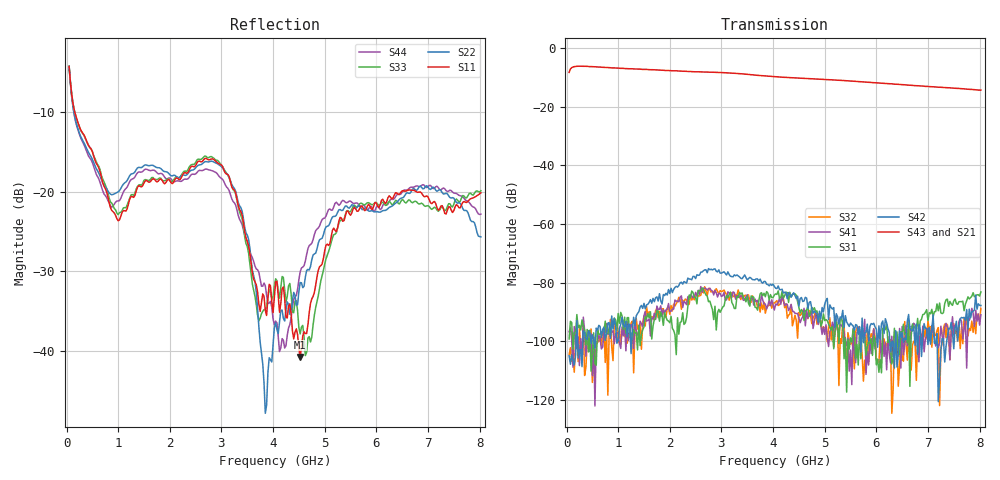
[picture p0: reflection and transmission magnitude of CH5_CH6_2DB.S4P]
!Agilent Technologies,E5071C,MY46316741,A.11.02
!Date: Mon Jun 01 10:40:18 2026
!Data & Calibration Information:
!1:CH5 INPUT 2:CH5 OUTPUT 3:CH6 INPUT 4:CH6 OUTPUT
!Freq	S11:SOLT4(ON)	S12:SOLT4(ON)	S13:SOLT4(ON)	S14:SOLT4(ON)
!	S21:SOLT4(ON)	S22:SOLT4(ON)	S23:SOLT4(ON)	S24:SOLT4(ON)
!	S31:SOLT4(ON)	S32:SOLT4(ON)	S33:SOLT4(ON)	S34:SOLT4(ON)
!	S41:SOLT4(ON)	S42:SOLT4(ON)	S43:SOLT4(ON)	S44:SOLT4(ON)
!PortZ  Port1:50+j0  Port2:50+j0  Port3:50+j0  Port4:50+j0
!Above PortZ is port z conversion or system Z0 setting when saving the data.
!When reading, reference impedance value at option line is always used.
# Hz S dB R 50
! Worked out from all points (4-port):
!   320 points, 50 MHz to 8.025 GHz, reference 50 ohm
!   strongest paths, dB at 50 MHz, 2.05 GHz, 4.05 GHz, 6.05 GHz, 8.025 GHz:
!     S43: -8.2, -7.7, -9.7, -11.8, -14.3
!     S21: -8.3, -7.9, -10.0, -12.1, -14.6
!     S42: -105.0, -83.4, -81.9, -94.8, -87.8
!     S31: -99.3, -95.7, -83.9, -110.6, -83.2
!     S41: -96.8, -89.0, -87.3, -96.8, -90.9
!     S32: -104.6, -89.7, -86.6, -107.3, -88.8
!   lowest |S11| = -40.7 dB at 4.525 GHz (marker M1), VSWR 1.02, Z = 49.8 - j0.882 ohm
!   |S11| at or under -10 dB: 160.2 MHz to end of sweep
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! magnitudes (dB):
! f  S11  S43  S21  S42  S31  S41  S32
! 50 MHz  -4.3  -8.2  -8.3  -105.0  -99.3  -96.8  -104.6
! 1 GHz  -23.6  -6.8  -7.0  -99.8  -90.6  -97.0  -100.5
! 3.15 GHz  -18.1  -8.4  -8.6  -77.3  -84.2  -83.6  -86.0
! 3.85 GHz  -34.9  -9.5  -9.7  -79.6  -84.8  -87.3  -90.5
! 4.525 GHz  -40.7  -10.2  -10.4  -85.5  -90.4  -93.7  -91.3
! 5.425 GHz  -22.5  -11.1  -11.3  -93.4  -117.4  -101.0  -107.2
! 8.025 GHz  -20.1  -14.3  -14.6  -87.8  -83.2  -90.9  -88.8
